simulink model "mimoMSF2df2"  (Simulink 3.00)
settings: Solver=ode45  StartTime=0.0  StopTime=50.0  RelTol=1e-3
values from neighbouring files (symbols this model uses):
  Disturb = Setpoint    [mimo_MSF1DF_sim.m]    (also in mimo_MSF2DF_sim.m)
  K = 1/kpd    [imc2pseucon.m]    (also in imc2pseudo.m)
  Satlb = temp1    [cback.m]    (also in imcmenu.m = str2num(satlbs))
  Satub = temp1    [cback.m]    (also in imcmenu.m = str2num(satubs))
  Setpoint = zeros(1,n)    [mimo_MSF1DF_sim.m]    (also in mimo_MSF2DF_sim.m)
undefined symbols (not defined in the file or in its folder): Ds, input_delay, Kdelay, Ksp, T
libraries: MIMO_lib x10, simulink3 x7

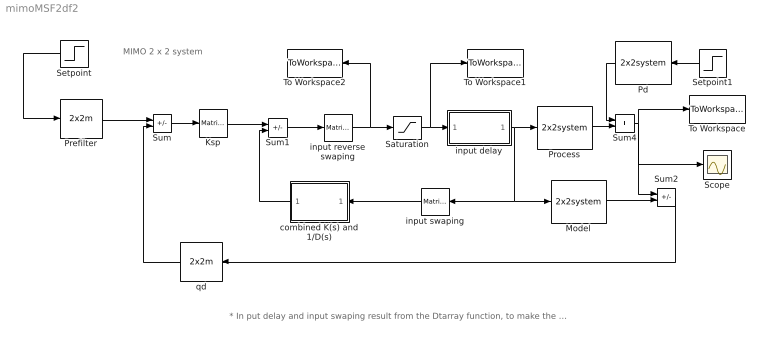
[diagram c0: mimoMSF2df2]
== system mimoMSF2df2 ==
  note: * In put delay and input swaping result from the Dtarray function, to make the system be able to be decoupled.
  note: MIMO 2 x 2 system
  Ksp : simulink3/Math/Matrix Gain  K=Ksp
  Model : MIMO_lib/2x2system  num=Mnum  den=Mden  dead=Mdead
  Pd : MIMO_lib/2x2system  Orientation=left  num=Pdnum  den=Pdden  dead=Pddead
  Prefilter : MIMO_lib/2x2m  num=prefilnum  den=prefilden
  Process : MIMO_lib/2x2system  num=Pnum  den=Pden  dead=Pdead
  Saturation : Saturate  UpperLimit=Satub  LowerLimit=Satlb
  Scope : Scope
  Setpoint : Step  Orientation=left  Time=0  Before=0  After=[Setpoint]  SampleTime=0
  Setpoint1 : Step  Orientation=left  Time=0  Before=0  After=[Disturb]  SampleTime=0
  Sum : Sum  Inputs=+-  SaturateOnIntegerOverflow=on
  Sum1 : Sum  Inputs=+-  SaturateOnIntegerOverflow=on
  Sum2 : Sum  Inputs=+-  SaturateOnIntegerOverflow=on
  Sum4 : Sum  Inputs=++  SaturateOnIntegerOverflow=on
  To Workspace : ToWorkspace  VariableName=yout  SampleTime=0  SaveFormat=Matrix
  To Workspace1 : ToWorkspace  VariableName=sat_effort  SampleTime=0  SaveFormat=Matrix
  To Workspace2 : ToWorkspace  VariableName=unsat_effort  SampleTime=0  SaveFormat=Matrix
  combined K(s) and 1/D(s) : Subsystem  Orientation=left  mask(ksds){Ksp=Ksp, Ds=Ds, Kdelay=Kdelay, K=K}
      mask prompts: Ds "D(s)"; Kdelay "Bdelay"; K "B*(s)"
  input delay : Subsystem  mask(input delay){input_delay=input_delay}
      mask prompts: input_delay "Input Delay (vector)"
  input reverse swaping : simulink3/Math/Matrix Gain  K=inv(T)
  input swaping : simulink3/Math/Matrix Gain  Orientation=left  K=T
  qd : MIMO_lib/2x2m  Orientation=left  num=qdnum  den=qdden
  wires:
  Ksp/1 -> Sum1/1
  combined K(s) and 1/D(s)/1(Out1) -> Sum1/2
  Sum/1 -> Ksp/1
  input swaping/1 -> combined K(s) and 1/D(s)/1(In1)
  Model/1 -> Sum2/2
  Process/1 -> Sum4/2
  Sum4/1 -> Sum2/1, To Workspace/1, Scope/1
  input reverse swaping/1 -> Saturation/1, To Workspace2/1
  Sum1/1 -> input reverse swaping/1
  input delay/1(Out1) -> Process/1, Model/1, input swaping/1
  Saturation/1 -> input delay/1(In1), To Workspace1/1
  Setpoint1/1 -> Pd/1
  Pd/1 -> Sum4/1
  qd/1 -> Sum/2
  Sum2/1 -> qd/1
  Prefilter/1 -> Sum/1
  Setpoint/1 -> Prefilter/1

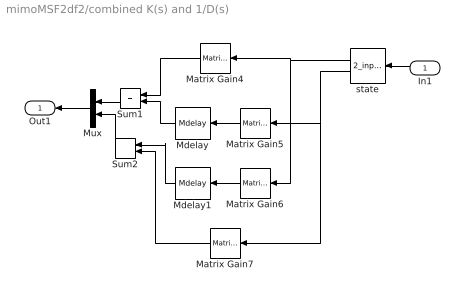
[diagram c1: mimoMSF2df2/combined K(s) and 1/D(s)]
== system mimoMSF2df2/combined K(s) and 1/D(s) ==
  In1 : Inport  Orientation=left  Port=1  PortWidth=-1  SampleTime=-1  DataType=auto
  Matrix Gain4 : simulink3/Math/Matrix Gain  Orientation=left  K="[zeros(1,length(Ds{1})-length(K{1,1}))  K{1,1}]"
  Matrix Gain5 : simulink3/Math/Matrix Gain  Orientation=left  K="[zeros(1,length(Ds{2})-length(K{1,2}))  K{1,2}]"
  Matrix Gain6 : simulink3/Math/Matrix Gain  Orientation=left  K="[zeros(1,length(Ds{1})-length(K{2,1}))  K{2,1}]"
  Matrix Gain7 : simulink3/Math/Matrix Gain  Orientation=left  K=[zeros(1,length(Ds{2})-length(K{2,2}) ) K{2,2}]
  Mdelay : MIMO_lib/Mdelay  Orientation=left  Mdelay=Kdelay(1,2)
  Mdelay1 : MIMO_lib/Mdelay  Orientation=left  Mdelay=Kdelay(2,1)
  Mux : Mux  Orientation=left  Inputs=2
  Sum1 : Sum  Orientation=left  Inputs=++  SaturateOnIntegerOverflow=on
  Sum2 : Sum  Orientation=left  Inputs=++  SaturateOnIntegerOverflow=on
  state : MIMO_lib/2_input_state  Orientation=left  Ds=Ds
  Out1 : Outport  Orientation=left  Port=1
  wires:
  Sum1/1 -> Mux/1
  Matrix Gain4/1 -> Sum1/1
  Mdelay/1 -> Sum1/2
  Matrix Gain5/1 -> Mdelay/1
  Sum2/1 -> Mux/2
  Matrix Gain6/1 -> Mdelay1/1
  Mdelay1/1 -> Sum2/1
  Matrix Gain7/1 -> Sum2/2
  Mux/1 -> Out1/1
  In1/1 -> state/1
  state/1 -> Matrix Gain4/1, Matrix Gain6/1
  state/2 -> Matrix Gain5/1, Matrix Gain7/1

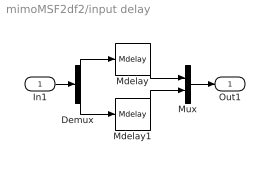
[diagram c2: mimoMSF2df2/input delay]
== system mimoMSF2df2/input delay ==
  In1 : Inport  Port=1  PortWidth=-1  SampleTime=-1  DataType=auto
  Demux : Demux  Outputs=2
  Mdelay : MIMO_lib/Mdelay  Mdelay=input_delay(1)
  Mdelay1 : MIMO_lib/Mdelay  Mdelay=input_delay(2)
  Mux : Mux  Inputs=2
  Out1 : Outport  Port=1
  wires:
  Mux/1 -> Out1/1
  In1/1 -> Demux/1
  Demux/1 -> Mdelay/1
  Demux/2 -> Mdelay1/1
  Mdelay/1 -> Mux/1
  Mdelay1/1 -> Mux/2
